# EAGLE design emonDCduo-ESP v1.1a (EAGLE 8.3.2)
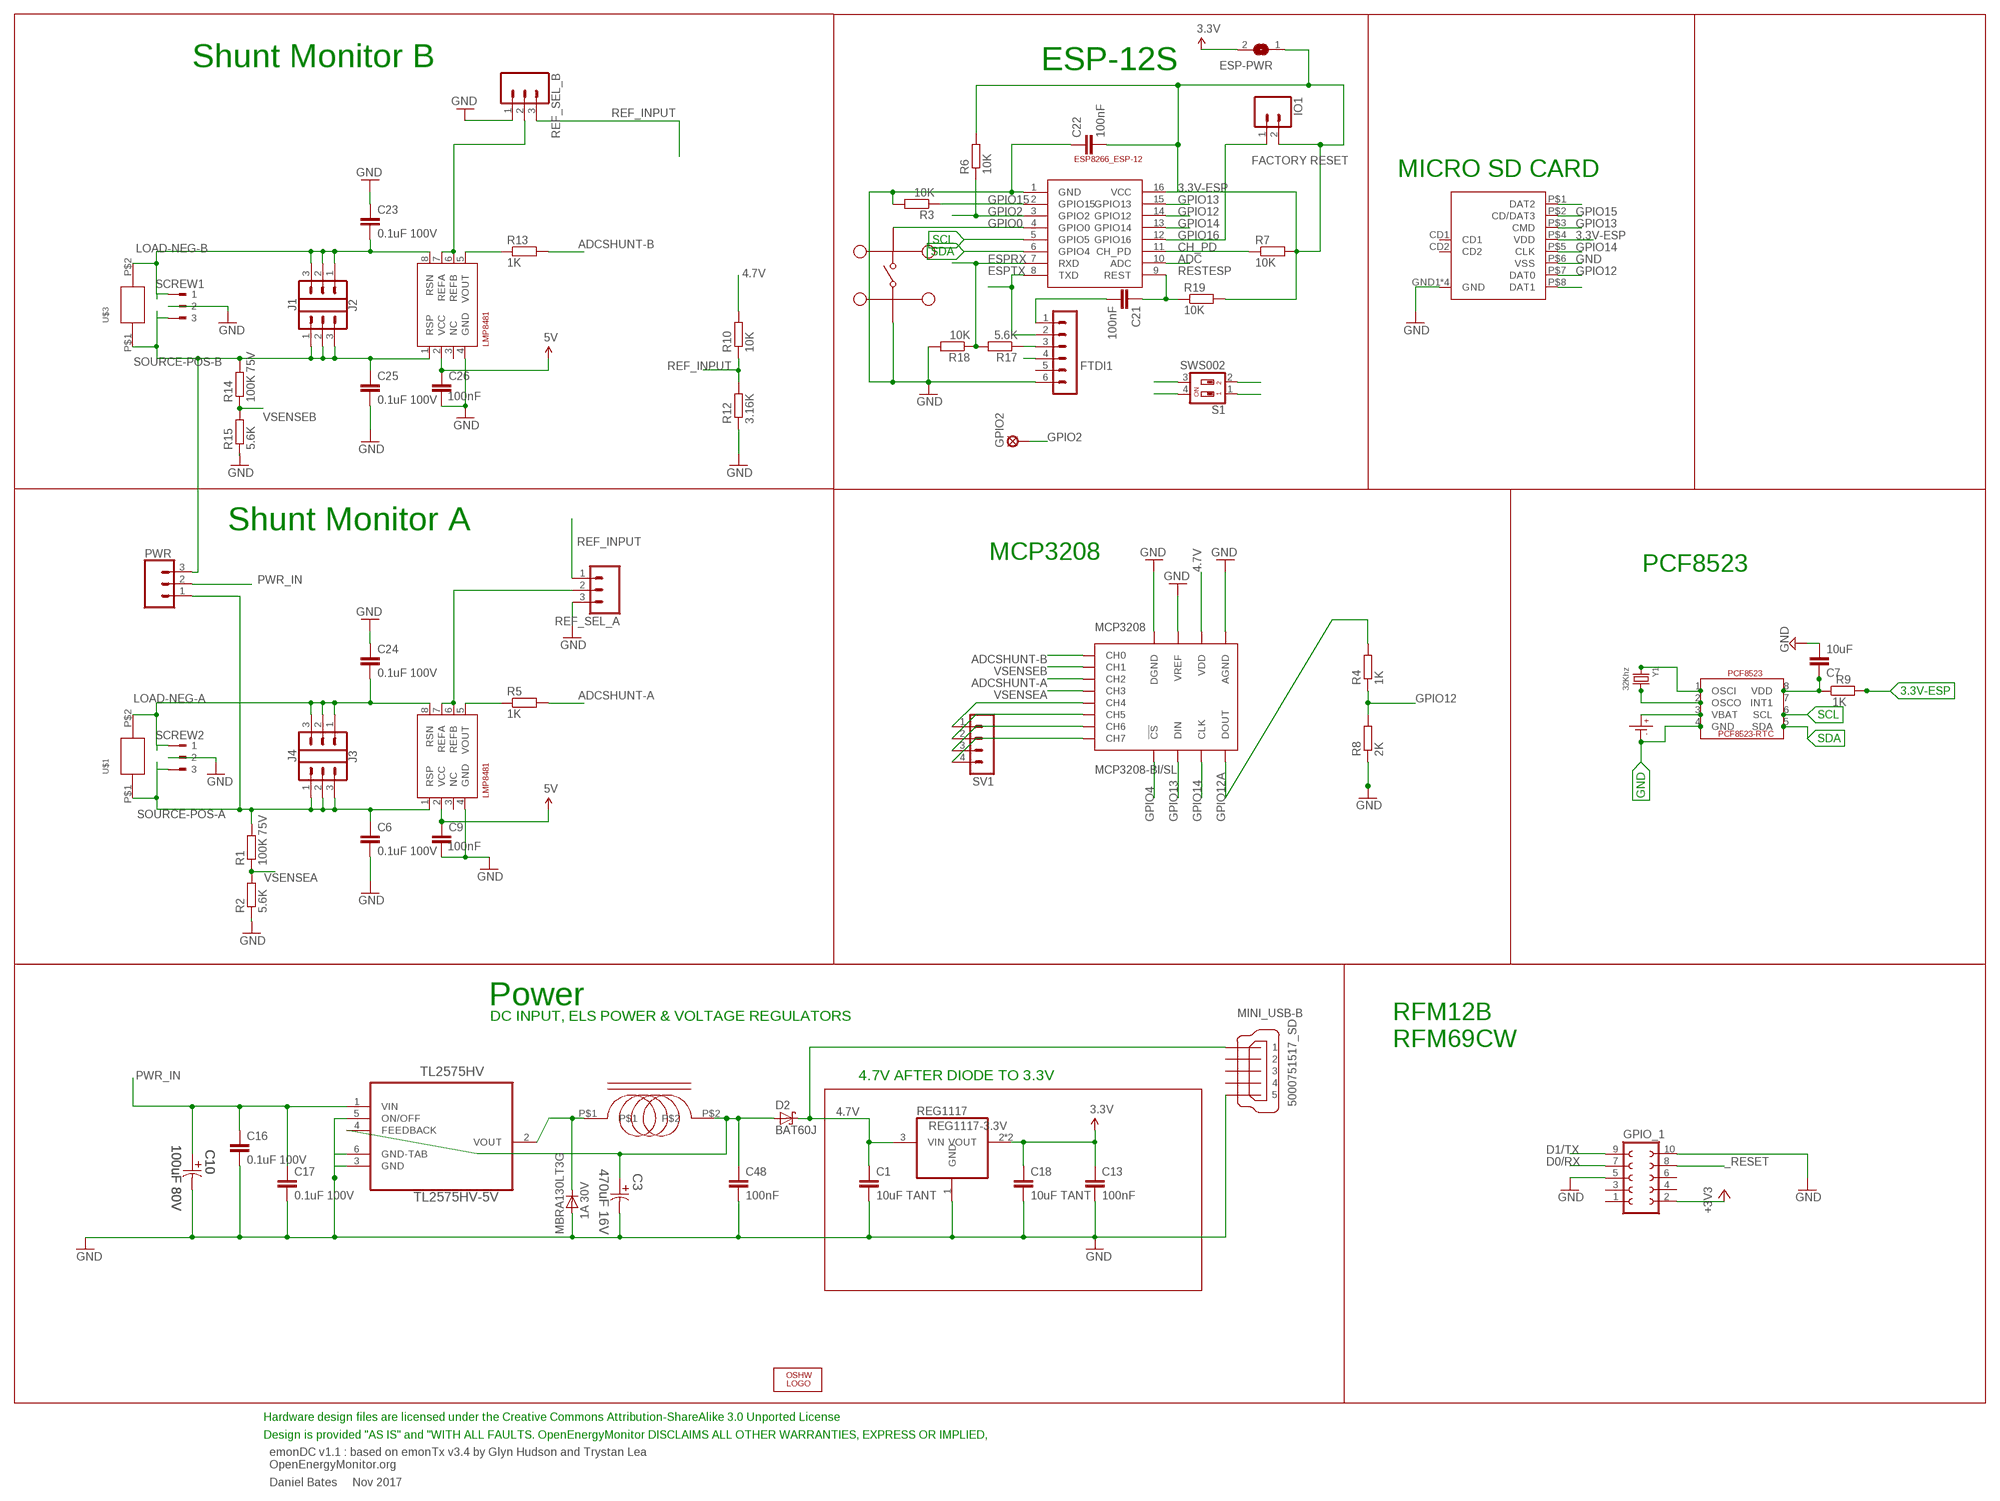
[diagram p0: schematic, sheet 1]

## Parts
C1  10uF TANT  C-EUC0603  [C0603]
C3  470uF 16V  EEE-FK1C471P-CASE-F  [CAPAE830X1050N]
C6  0.1uF 100V  C-EUC0603  [C0603]
C7  10uF  C-EUC0603  [C0603]
C9  100nF  C-EUC0603  [C0603]
C10  100uF 80V  EEV-FK1K101Q-CASE-H13  [CAPAE1350X1400N]
C13  100nF  C-EUC0603  [C0603]
C16  0.1uF 100V  C-EUC0603  [C0603]
C17  0.1uF 100V  C-EUC0603  [C0603]
C18  10uF TANT  C-EUC0603  [C0603]
C21  100nF  C-EUC0603  [C0603]
C22  100nF  C-EUC0603  [C0603]
C23  0.1uF 100V  C-EUC0603  [C0603]
C24  0.1uF 100V  C-EUC0603  [C0603]
C25  0.1uF 100V  C-EUC0603  [C0603]
C26  100nF  C-EUC0603  [C0603]
C48  100nF  C-EUC0603  [C0603]
D1  MBRA130LT3G  [DO-214]
D2  BAT60J  [SOD323_ST]
ESP-12  ESP8266_ESP-12  [ESP8266-ESP12]
ESP-PWR  SJ  [SJ]
FTDI1  FTDI-ESP  MA06-1  [MA06-1]
GPIO2  LSP11  [LSP11]
GPIO_1  FE05-2  [FE05-2]
I1  330uH  SRR0603-331KL  [SRR0603-331KL]
IO1  M02PTH  [1X02]
J1  CONN_03  [1X03]
J2  CONN_03  [1X03]
J3  CONN_03  [1X03]
J4  CONN_03  [1X03]
LOGO1  OSHW_LOGO_6MILX0200-NT  [OSHW_6X200_NOTEXT]
MC2  MC32882  [SWITCH_TACT_MULTICOMP]
MCP3208  MCP3208-BI/SL  [SOIC16]
MINI_USB-B  5000751517_SD  [5000751517_SD]
PCF8523  PCF8523_RTC  [SOIC_8]
PWR  CONN_03  [1X03]
R1  100K 75V  R-EU_R0603  [R0603]
R2  5.6K  R-EU_R0603  [R0603]
R3  10K  R-EU_R0603  [R0603]
R4  1K  R-EU_R0603  [R0603]
R5  1K  R-EU_R0603  [R0603]
R6  10K  R-EU_R0603  [R0603]
R7  10K  R-EU_R0603  [R0603]
R8  2K  R-EU_R0603  [R0603]
R9  1K  R-EU_R0603  [R0603]
R10  10K  R-EU_R0603  [R0603]
R12  3.16K  R-EU_R0603  [R0603]
R13  1K  R-EU_R0603  [R0603]
R14  100K 75V  R-EU_R0603  [R0603]
R15  5.6K  R-EU_R0603  [R0603]
R17  5.6K  R-EU_R0603  [R0603]
R18  10K  R-EU_R0603  [R0603]
R19  10K  R-EU_R0603  [R0603]
REF_SEL_A  2212S-02SG-85  CONN_03  [1X03]
REF_SEL_B  2212S-02SG-85  CONN_03  [1X03]
REG1117  REG1117-3.3V  REG1117-VOUT4  [SOT223]
S1  SWS002  [SMS-002]
SCREW1  180-3  [180-3]
SCREW2  180-3  [180-3]
SHUNTMON-A  LMP8481  LMP8481-H  [S-PDSO-G08]
SHUNTMON-B  LMP8481  LMP8481-H  [S-PDSO-G08]
SV1  MA04-1  [MA04-1]
TL2575HV  TL2575HV-5V  TL2575HV-05IKTTR  [TO-263]
U$1  EBW_SERIES_10.5MM  [EBW_SERIES_10.5MM]
U$2  MOLEX_MICRO_SD_1040310811  [MOLEX_MICROSD_EXPOSED]
U$3  EBW_SERIES_10.5MM  [EBW_SERIES_10.5MM]
U$18  CR1220SMD  [CR1220SMD]
Y1  32Khz  CRYSTAL8X3.8SMT  [CRYSTAL_8X3.8]

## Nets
3.3V: C13.1 C18.1 ESP-PWR.2 GPIO_1.2 REG1117.2(VOUT) REG1117.4(VOUT) ; supply symbol labelled +3V3
3.3V-ESP: C22.2 ESP-12.16(VCC) ESP-PWR.1 IO1.2 R6.2 R7.2 R9.2 R19.2 U$2.P$4(VDD)
4.7V [power]: C1.1 C9.1 C26.1 D2.C FTDI1.4 MCP3208.16(VDD) MINI_USB-B.VBUS R10.2 REG1117.3(VIN) SHUNTMON-A.2(VCC) SHUNTMON-B.2(VCC) ; supply symbol labelled 5V
5.0V [power]: C3.1 C48.1 D2.A I1.P$2 TL2575HV.4(FEEDBACK)
_RESET: GPIO_1.8
ADC: ESP-12.10(ADC)
ADCSHUNT-A: MCP3208.3(CH2) R5.2
ADCSHUNT-B: MCP3208.1(CH0) R13.2
CH_PD: ESP-12.11(CH_PD) R7.1
D0/RX: GPIO_1.7 S1.2
D1/TX: GPIO_1.9 S1.1
ESPRX: ESP-12.7(RXD) R17.2 R18.1 S1.4
ESPTX: ESP-12.8(TXD) FTDI1.2 S1.3
GND [thin_power]: C1.2 C3.2 C6.2 C7.2 C9.2 C10.2 C13.2 C16.2 C17.2 C18.2 C22.1 C23.1 C24.1 C25.2 C26.2 C48.2 D1.P$2(A) ESP-12.1(GND) FTDI1.6 GPIO_1.5 GPIO_1.10 MC2.P$1 MC2.P$2 MCP3208.9(DGND) MCP3208.14(AGND) MCP3208.15(VREF) MINI_USB-B.GND1 MINI_USB-B.GND2 MINI_USB-B.GND3 PCF8523.4(GND) R2.1 R3.2 R8.1 R12.1 R15.1 R18.2 REF_SEL_A.3 REF_SEL_B.1 REG1117.1(GND) SCREW1.2 SCREW2.2 SHUNTMON-A.4(GND) SHUNTMON-B.4(GND) TL2575HV.3(GND) TL2575HV.5(ON/OFF) TL2575HV.6(GND-TAB) U$2.GND1(GND) U$2.GND2(GND) U$2.GND3(GND) U$2.GND4(GND) U$2.P$6(VSS) U$18.P-(P$-)
GPIO0: ESP-12.4(GPIO0) MC2.P$3 MC2.P$4
GPIO2: ESP-12.3(GPIO2) GPIO2.MP R6.1
GPIO4: MCP3208.10(!CS)
GPIO12: ESP-12.14(GPIO12) R4.1 R8.2 U$2.P$7(DAT0)
GPIO12A: MCP3208.12(DOUT) R4.2
GPIO13: ESP-12.15(GPIO13) MCP3208.11(DIN) U$2.P$3(CMD)
GPIO14: ESP-12.13(GPIO14) MCP3208.13(CLK) U$2.P$5(CLK)
GPIO15 [thin_power]: ESP-12.2(GPIO15) R3.1 U$2.P$2(CD/DAT3)
GPIO16: ESP-12.12(GPIO16) IO1.1
IND: D1.P$1(C) I1.P$1 TL2575HV.2(VOUT)
LOAD-NEG-A: C24.2 J4.1 J4.2 J4.3 SCREW2.1 SHUNTMON-B.8(RSN) U$1.P$2
LOAD-NEG-B: C23.2 J1.1 J1.2 J1.3 SCREW1.1 SHUNTMON-A.8(RSN) U$3.P$2
N$1: MCP3208.5(CH4) SV1.1
N$3: MCP3208.6(CH5) SV1.2
N$4: R13.1 SHUNTMON-A.5(VOUT)
N$5: MCP3208.7(CH6) SV1.3
N$6: R5.1 SHUNTMON-B.5(VOUT)
N$7: U$2.P$1(DAT2)
N$9: MCP3208.8(CH7) SV1.4
N$10: C7.1 PCF8523.8(VDD) R9.1
N$30: C21.2 FTDI1.1
N$32: U$2.P$8(DAT1)
N$36: FTDI1.3 R17.1
N$43: PCF8523.3(VBAT) U$18.P+(P$+)
N$44: PCF8523.2(OSCO) Y1.P$4
N$45: PCF8523.1(OSCI) Y1.P$1
PWR_IN: C10.1 C16.1 C17.1 PWR.2 TL2575HV.1(VIN)
REF_A_INPUT [thin_power]: REF_SEL_A.2 SHUNTMON-B.6(REFB) SHUNTMON-B.7(REFA)
REF_B_INPUT: REF_SEL_B.2 SHUNTMON-A.6(REFB) SHUNTMON-A.7(REFA)
REF_INPUT: R10.1 R12.2 REF_SEL_A.1 REF_SEL_B.3
RESTESP: C21.1 ESP-12.9(REST) R19.1
SCL: ESP-12.5(GPIO5) PCF8523.6(SCL)
SDA: ESP-12.6(GPIO4) PCF8523.5(SDA)
SOURCE-POS-A: C6.1 J3.1 J3.2 J3.3 PWR.1 R1.2 SCREW2.3 SHUNTMON-B.1(RSP) U$1.P$1
SOURCE-POS-B: C25.1 J2.1 J2.2 J2.3 PWR.3 R14.2 SCREW1.3 SHUNTMON-A.1(RSP) U$3.P$1
VSENSEA: MCP3208.4(CH3) R1.1 R2.2
VSENSEB: MCP3208.2(CH1) R14.1 R15.2
Unconnected: FTDI1.5 GPIO_1.1 GPIO_1.3 GPIO_1.4 GPIO_1.6 MINI_USB-B.D+ MINI_USB-B.D- MINI_USB-B.ID PCF8523.7(INT1) SHUNTMON-A.3(NC) SHUNTMON-B.3(NC) U$2.CD1 U$2.CD2

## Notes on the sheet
- Shunt Monitor B | ESP-12S
- FACTORY RESET
- MICRO SD CARD
- Shunt Monitor A
- MCP3208
- PCF8523
- Power
- DC INPUT, ELS POWER & VOLTAGE REGULATORS
- RFM12B
  RFM69CW
- 4.7V AFTER DIODE TO 3.3V
- Hardware design files are licensed under the Creative Commons Attribution-ShareAlike 3.0 Unported License
- Design is provided "AS IS" and "WITH ALL FAULTS. OpenEnergyMonitor DISCLAIMS ALL OTHER WARRANTIES, EXPRESS OR IMPLIED,
- emonDC v1.1 : based on emonTx v3.4 by Glyn Hudson and Trystan Lea
  OpenEnergyMonitor.org
- Daniel Bates     Nov 2017

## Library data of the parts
C1 C7 C13 C16-C18 C21 C22 C48 = rcl:C-EU: CAPACITOR, European symbol
C3 = Panasonic-EEEFK_EEEFP:EEE-: Aluminum Electrolytic Capacitors,Surface Mount Type; MPN: EEE-FK1C471P; OC_FARNELL: 9695710; OC_NEWARK: 96K9385; PACKAGE: CASE-F; SUPPLIER: PANASONIC; TOLERANCE: ±20 %; VALUE: 470UF; VOLTAGERATING: 16V
C6 C9 C23-C26 = rcl:C-EU: CAPACITOR, European symbol; MPN: C1608X7S2A104K080AB
C10 = Panasonic-EEE-EEV-EEF-ECQ:EEV-: Aluminum Electrolytic Capacitors,Surface Mount Type; MPN: EEVFK1K101Q; OC_FARNELL: 9696113; OC_NEWARK: 96K9484; SUPPLIER: PANASONIC; TOLERANCE: ±20 %; VALUE: 100UF; VOLTAGERATING: 80V
D1 = CASE 403D Diode:MBRA130LT3G: Fast switching diode; MF: ON SEMICONDUCTOR; MPN: MBRA130LT3G; OC_FARNELL: 9555978
D2 = diode:BAT60J: Schottky barrier diode
ESP-12 = ESP8266-ESP12:ESP8266_ESP-12
ESP-PWR = jumper:SJ: SMD solder JUMPER
FTDI1 = JeeLabs:MA06-1: PIN HEADER
GPIO2 = solpad:LSP11: SOLDER PAD
GPIO_1 = con-lsta:FE05-2: FEMALE HEADER; OC_FARNELL: unknown; OC_NEWARK: unknown
I1 = SRR0603-331KL:SRR0603-331KL: SRR0603-331KL; INDUCTANCE: 330uH; MF: BOURNS; MPN: SRR0603-331KL; OC_FARNELL: 2333890
IO1 = SparkFun:M02: Header 2
J1-J4 PWR = SparkFun-Connectors:CONN_03: Multi connection point. Often used as Generic Header-pin footprint for 0.1 inch spaced/style header connections On any of the 0.1 inch spaced packages, you can populate with these: Break Away Headers - Straight (PRT-00116) Break Away Male Headers - Right Angle (PRT-00553) Female Headers (PRT-00115)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
LOGO1 = ohw-logo:OSHW_LOGO_6MIL; OC_FARNELL: unknown
MC2 = multicomp tact switch:MC32882
MCP3208 = MCP3208:MCP3208
MINI_USB-B = 5000751517_sd:5000751517_SD
PCF8523 = IotaWatt_parts:PCF8523_RTC: PCF8523-RTC SOIC-8
R1 R14 = rcl:R-EU_: RESISTOR, European symbol; MPN: MCWR06X1003FTL
R2 R4 R8 R15 = rcl:R-EU_: RESISTOR, European symbol; MPN: MCWR06X5901FTL
R3 R5-R7 R9 R10 R12 R13 R17-R19 = rcl:R-EU_: RESISTOR, European symbol
REF_SEL_A REF_SEL_B = SparkFun-Connectors:CONN_03: Multi connection point. Often used as Generic Header-pin footprint for 0.1 inch spaced/style header connections On any of the 0.1 inch spaced packages, you can populate with these: Break Away Headers - Straight (PRT-00116) Break Away Male Headers - Right Angle (PRT-00553) Female Headers (PRT-00115)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; MF: MULTICOMP; MPN: 2212S-02SG-85; OC_FARNELL: 1593458
REG1117 = burr-brown:REG1117-VOUT4: 800mA and 1A Low Dropout (LDO) Positive Regulator 1.8V, 2.5V, 2.85V, 3.3V, 5V, and Adj; MF: TEXAS INSTRUMENTS; MPN: REG1117; OC_FARNELL: 1097566; OC_NEWARK: 14P6981
S1 = smd-special:SWS002: SMD Dip Switch 2 pol.
SCREW1 SCREW2 = con-weidmueller-sl35:180-3: WEIDMUELLER CLAMP CONNECTOR; OC_FARNELL: unknown; OC_NEWARK: unknown
SHUNTMON-A = lmp8481b:LMP8481: LMP8481MM-H/NOPB 100V/V; MF: TEXAS INSTRUMENTS; MPN: LMP8481MME-S/NOPB; OC_FARNELL: 2322044
SHUNTMON-B = lmp8481b:LMP8481: LMP8481MM-H/NOPB 100V/V; MF: TEXAS INSTRUMENTS; MPN: LMP8481MME-H/NOPB; OC_FARNELL: 2322044
SV1 = con-lstb:MA04-1: PIN HEADER; OC_FARNELL: unknown; OC_NEWARK: unknown
TL2575HV = TL2575HV:TL2575HV; MF: TEXAS INSTRUMENTS; MPN: LM2575HVS-15/NOPB; OC_FARNELL: 2492609
U$1 U$3 = EBW series shunt:EBW_SERIES_10.5MM
U$2 = MOLEX MICRO SD [exposed pins]:MOLEX_MICRO_SD_1040310811
U$18 = IotaWatt_parts:CR1220SMD: CR1220 Battery SMD
Y1 = microbuilder:CRYSTAL: Crystals

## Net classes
2 thin_power: width 0.254 mm

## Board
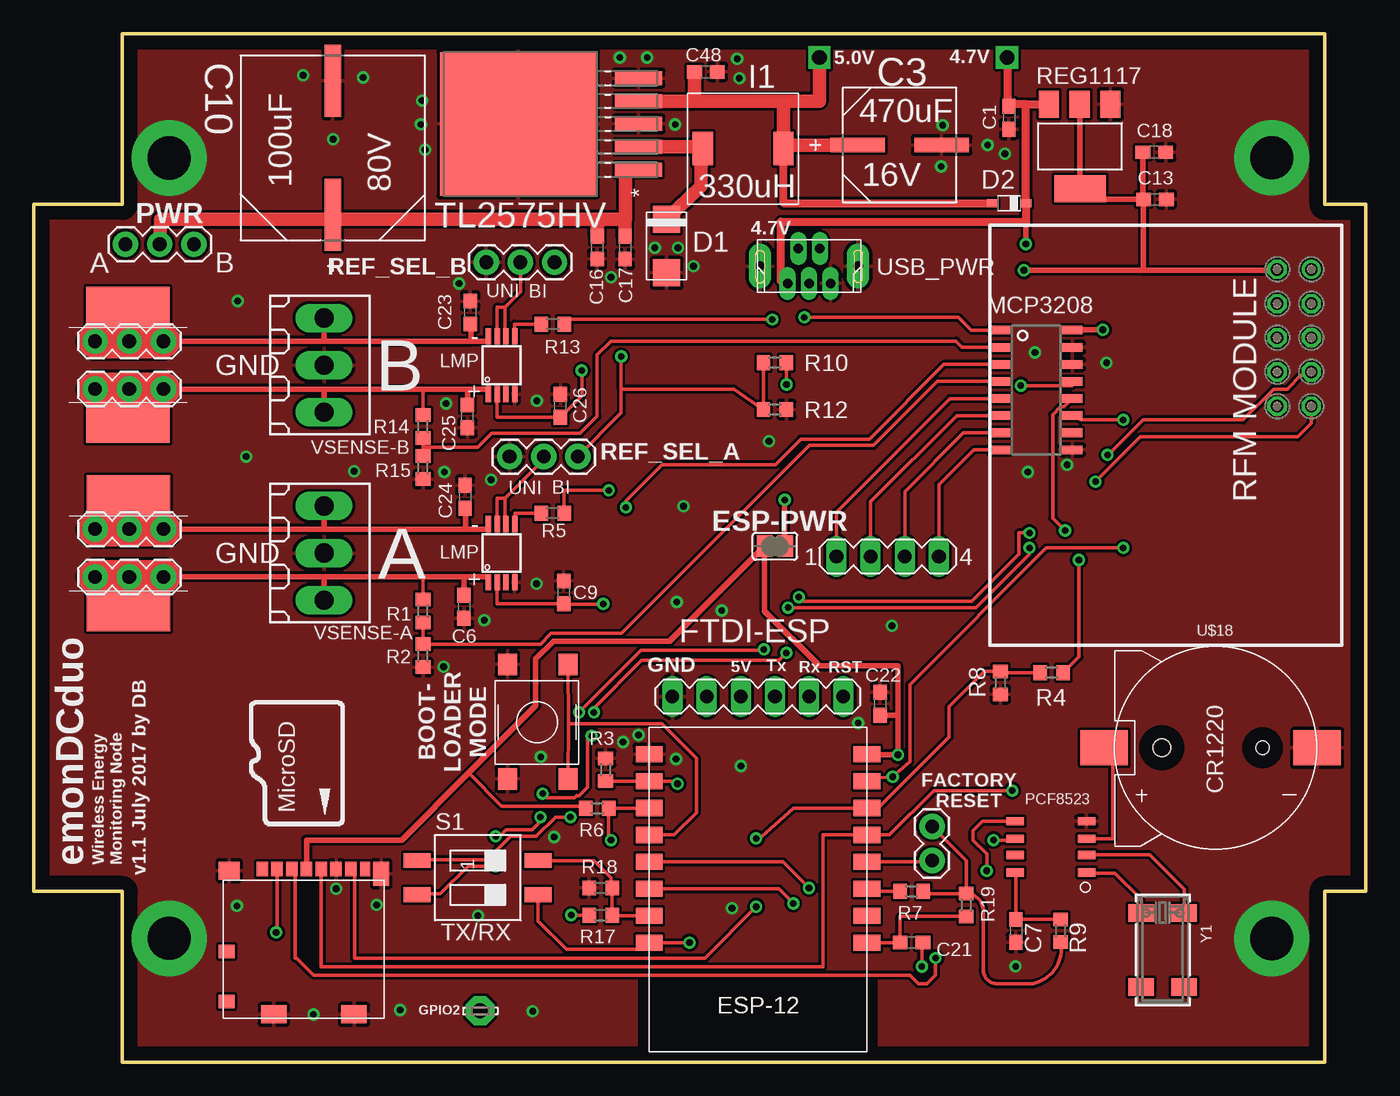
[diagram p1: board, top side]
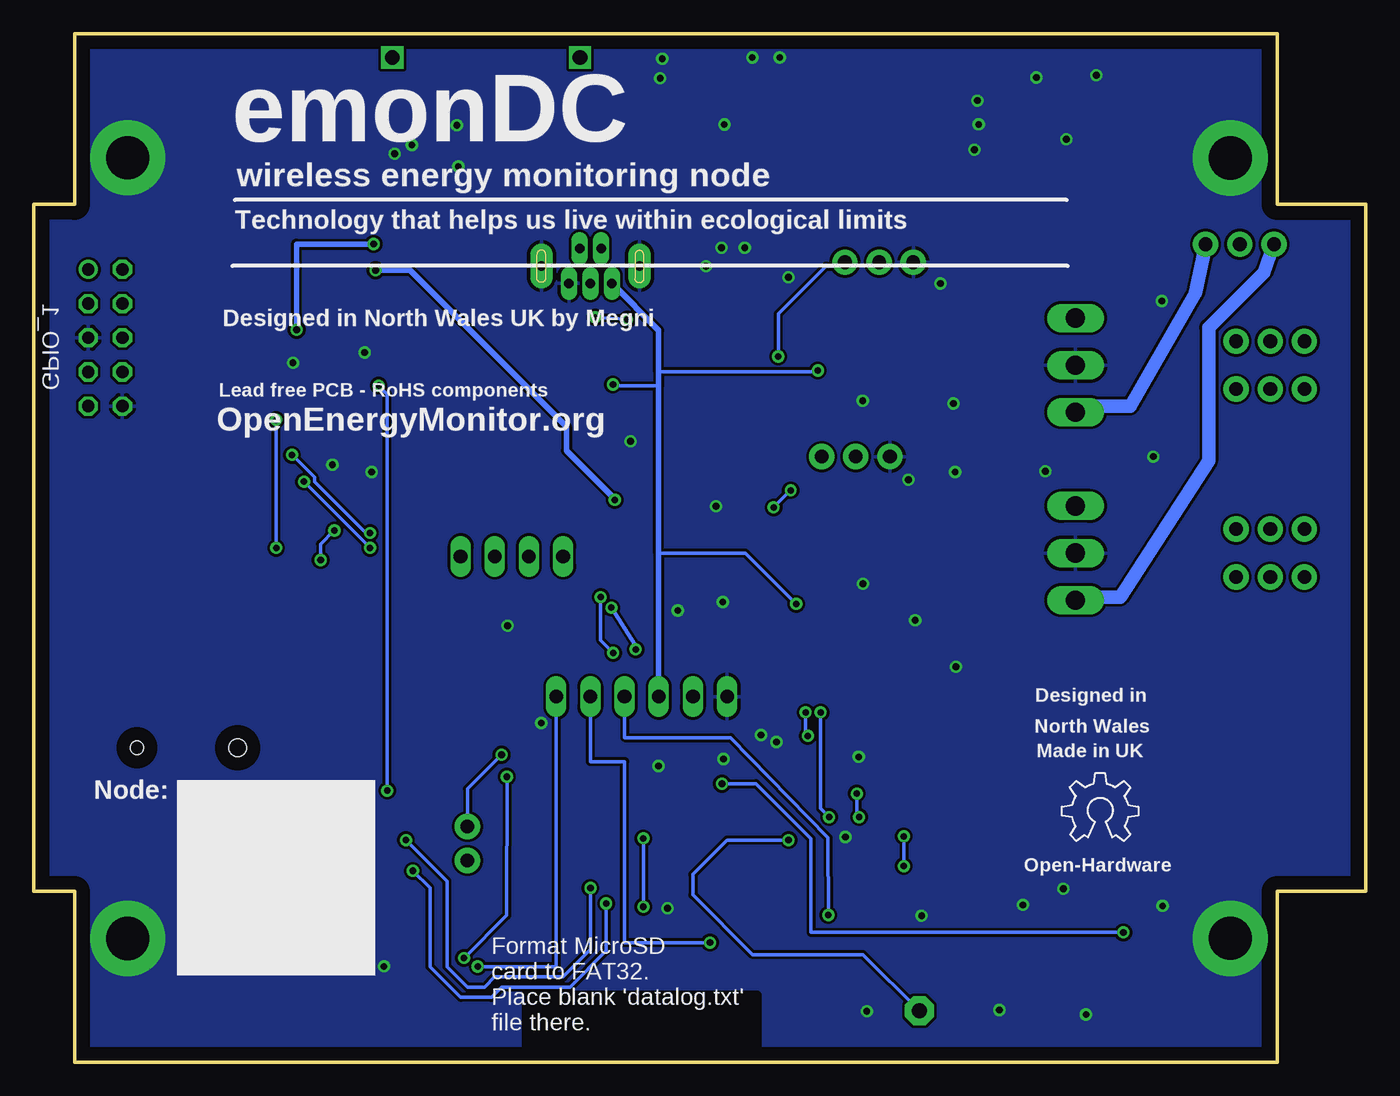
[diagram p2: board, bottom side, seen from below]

Size 99.06 x 76.45 mm. Coordinates in mm from the lower left corner, seen from the top.
Outline: 6.6,63.75 6.6,76.45 96.01,76.45 96.01,63.75 99.06,63.75 99.06,12.7 96.01,12.7 96.01,0 6.6,0 6.6,12.7 0,12.7 0,63.75 6.6,63.75
Copper layers (1*16): Top 0.035mm / dielectric 1.5mm / Bottom 0.035mm
Design rules "default *": minimum track width 10mil, minimum drill 19mil, track to track 8mil, track to pad 8mil, pad to pad 8mil, via to via 8mil, smd to smd 8mil, copper to edge 40mil, drill to drill 8mil, minimum pad ring 10mil, minimum via ring 8mil, stop-mask expansion 4mil, vias tented up to drill 0mil, thermal gap 10mil
tRestrict: area 45.2,1 to 62.5,6.1
bRestrict: area 45.2,1 to 62.5,5.1

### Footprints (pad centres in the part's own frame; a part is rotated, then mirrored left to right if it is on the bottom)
C0603 = smd 1.1 x 1: 1 -0.85,0; 2 0.85,0
CAPAE830X1050N = smd 4.064 x 1.092: 1 -3.124,0; 2 3.124,0
CAPAE1350X1400N = smd 5.359 x 1.194: 1 -4.978,0; 2 4.978,0
DO-214 = smd 2 x 2: P$1 -2,0; P$2 2,0
SOD323_ST = smd 0.8 x 0.6: A 1.25,0; C -1.25,0
ESP8266-ESP12 = smd 2 x 1.2: 1 16.2,2; 2 16.2,4; 3 16.2,6; 4 16.2,8; 5 16.2,10; 6 16.2,12; 7 16.2,14; 8 16.2,16; 9 0,16; 10 0,14; 11 0,12; 12 0,10; 13 0,8; 14 0,6; 15 0,4; 16 0,2
SJ = smd 1.168 x 1.6: 1 -0.762,0; 2 0.762,0
MA06-1 = drill 1.016 long: 1 0,0; 2 2.54,0; 3 5.08,0; 4 7.62,0; 5 10.16,0; 6 12.7,0
LSP11 = drill 1.118 pad 2.159 octagon: MP 0,0
FE05-2 = drill 0.914: 1 -5.08,1.27 | drill 0.914 octagon: 2 -5.08,-1.27; 3 -2.54,1.27; 4 -2.54,-1.27; 5 0,1.27; 6 0,-1.27; 7 2.54,1.27; 8 2.54,-1.27; 9 5.08,1.27; 10 5.08,-1.27
SRR0603-331KL = smd 1.5 x 2.5: P$1 -3,0; P$2 3,0
1X02 = drill 1.016 pad 1.88: 1 0,0; 2 2.54,0
1X03 = drill 1.016 pad 1.88: 1 0,0; 2 2.54,0; 3 5.08,0
SWITCH_TACT_MULTICOMP = smd 1.6 x 1.4: P$1 -1.1,5.3; P$2 7.4,5.3; P$3 -1.1,0.8; P$4 7.4,0.8
SOIC16 = smd 0.635 x 1.524: 1 -4.445,-2.695; 2 -3.175,-2.695; 3 -1.905,-2.695; 4 -0.635,-2.695; 5 0.635,-2.695; 6 1.905,-2.695; 7 3.175,-2.695; 8 4.445,-2.695; 9 4.445,2.695; 10 3.175,2.695; 11 1.905,2.695; 12 0.635,2.695; 13 -0.635,2.695; 14 -1.905,2.695; 15 -3.175,2.695; 16 -4.445,2.695
5000751517_SD = drill 0.7 pad 1.016 long: D+ 0,-1.3; D- -0.8,1.3; GND1 1.6,-1.3; ID 0.8,1.3; VBUS -1.6,-1.3 | drill 0.7 pad 1.676 long: GND2 3.65,0; GND3 -3.65,0
SOIC_8 = smd 1.3 x 0.6: 1 -2.6,1.9; 2 -2.6,0.6; 3 -2.6,-0.6; 4 -2.6,-1.9; 5 2.7,-1.9; 6 2.7,-0.6; 7 2.7,0.6; 8 2.7,1.9
R0603 = smd 1 x 1.1: 1 -0.85,0; 2 0.85,0
SOT223 = smd 1.499 x 2.007: 1 -2.261,-3.15; 2 0.025,-3.15; 3 2.311,-3.15 | smd 3.81 x 2.007: 4 0,3.15
SMS-002 = smd 1.092 x 2.007: 1 -1.27,-4.496; 2 1.27,-4.496; 3 1.27,4.496; 4 -1.27,4.496
180-3 = drill 1.422 long: 1 -3.5,0; 2 0,0; 3 3.5,0
S-PDSO-G08 = smd 0.4 x 1.2: 1 -0.975,-2.157; 2 -0.325,-2.157; 3 0.325,-2.157; 4 0.975,-2.157; 5 0.975,2.157; 6 0.325,2.157; 7 -0.325,2.157; 8 -0.975,2.157
MA04-1 = drill 1.016 long: 1 -3.81,0; 2 -1.27,0; 3 1.27,0; 4 3.81,0
TO-263 = smd 1.041 x 3.505: 1 -3.404,-8.788; 2 -1.702,-8.788; 3 0,-8.788; 4 1.702,-8.788; 5 3.404,-8.788 | smd 10.668 x 11.659: 6 0,0.152
EBW_SERIES_10.5MM = smd 3 x 6.2: P$1 -4.3,0; P$2 4.3,0
MOLEX_MICROSD_EXPOSED = smd 1.195 x 1.005: CD1 5.349,0.435; CD2 5.349,4.135 | smd 1.907 x 1.348: GND1 -4.112,5.104; GND2 1.853,5.104 | smd 1.17 x 1.793: GND3 -6.134,-5.352 | smd 1.551 x 1.348: GND4 5.167,-5.577 | smd 0.851 x 1.092: P$1 2.707,-5.703; P$2 1.617,-5.703; P$3 0.522,-5.699; P$4 -0.586,-5.701; P$5 -1.676,-5.703; P$6 -2.769,-5.703; P$7 -3.875,-5.701 | smd 0.749 x 1.092: P$8 -4.935,-5.701
CR1220SMD = smd 3.54 x 2.6: P+ 8.3,0; P- -7.55,0 | hole 1: -3.5,0 | hole 1.3: 4,0
CRYSTAL_8X3.8 = smd 1.3 x 1.9: P$1 -2.75,-1.6; P$2 2.75,-1.6; P$3 2.75,1.6; P$4 -2.75,1.6

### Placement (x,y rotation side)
C1  72.52,70.21 270 top
C3  64.39,68.17 0 top
C6  32,33.86 270 top
C7  73.04,9.76 270 top
C9  39.42,34.93 90 top
C10  22.25,67.96 90 top
C13  83.38,64.13 0 top
C16  41.9,60.55 270 top
C17  43.97,60.55 270 top
C18  83.32,67.64 0 top
C21  65.28,8.89 0 top
C22  62.94,26.64 270 top
C23  32.46,55.73 270 top
C24  32.08,42.04 270 top
C25  32.26,48.01 270 top
C26  39.17,48.8 90 top
C48  49.99,73.61 0 top
D1  47.06,60.67 270 top
D2  72.53,63.85 180 top
ESP-12  61.98,24.89 180 top
ESP-PWR  55.12,38.35 0 top
FTDI1  60.2,27.18 180 top
GPIO2  33.21,3.81 0 top
GPIO_1  93.73,53.85 270 top
I1  52.76,67.91 0 top
IO1  66.8,14.99 90 top
J1  4.57,53.59 0 top
J2  4.57,50.04 0 top
J3  4.57,36.07 0 top
J4  4.57,39.62 0 top
LOGO1  22.6,16.43 0 bottom
MC2  40.53,22.17 90 top
MCP3208  74.54,49.96 270 top
MINI_USB-B  57.66,59.18 0 top
PCF8523  75.69,16 180 top
PWR  6.84,60.8 0 top
R1  28.96,33.53 90 top
R2  28.96,30.23 90 top
R3  42.53,21.74 90 top
R4  75.69,28.96 0 top
R5  38.6,40.81 0 top
R6  41.91,18.87 180 top
R7  65.28,12.7 0 top
R8  71.88,28.19 90 top
R9  76.36,9.77 270 top
R10  55.12,52 0 top
R12  55.12,48.51 180 top
R13  38.61,54.86 0 top
R14  28.96,47.24 90 top
R15  28.96,44.2 90 top
R17  42.16,10.92 0 top
R18  42.16,12.95 180 top
R19  69.34,11.68 90 top
REF_SEL_A  40.47,45.01 180 top
REF_SEL_B  33.65,59.46 0 top
REG1117  77.8,68.07 180 top
S1  33.02,13.72 270 top
SCREW1  21.59,51.82 270 top
SCREW2  21.59,37.85 270 top
SHUNTMON-A  34.8,51.82 0 top
SHUNTMON-B  34.8,37.85 0 top
SV1  63.5,37.59 0 top
TL2575HV  36.19,69.74 90 top
U$1  7.05,37.82 90 top
U$2  19.71,8.66 180 top
U$3  7.02,51.83 90 top
U$18  87.88,23.37 180 top
Y1  83.95,8.35 270 top

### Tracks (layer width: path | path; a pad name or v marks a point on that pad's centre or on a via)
3.3V  (via drill 0.5)
  Top 0.254: 55.94,38.39 ESP-PWR.2 | 92.46,58.86 GPIO_1.2
  Top 0.406: REG1117.2 77.76,71.22 | 82.51,58.86 92.46,58.86 | 82.51,58.86 v73.63,58.86 | REG1117.4 78.6,64.13 C13.1 | C13.1 82.47,64.18 C18.1 | C13.1 82.51,64.11 82.51,58.86 | v55.84,41.8 55.84,38.49 55.94,38.39
  Bottom 0.406: v73.63,58.86 71.06,58.86 59.44,47.24 59.44,45.45 55.87,41.89 55.87,41.83 v55.84,41.8
3.3V-ESP  (via drill 0.5)
  Top 0.254: R7.2 66.13,12.53 R19.2 | R6.2 40.89,19.04 34.81,19.04 32.35,21.5 | IO1.2 69.34,14.99 R19.2 | R19.2 arc-90 70.61,11.26 70.61,6.86 arc90 71.63,5.84 74.29,5.84 arc90 R9.2
  Top 0.406: 64.26,25.91 64.26,29.46 58.42,29.46 54.36,33.53 ESP-PWR.1 47.29,31.28 38.65,31.28 37.34,29.97 37.34,26.49 32.35,21.5 27.35,16.51 20.3,16.51 U$2.P$4 | 64.26,25.91 v64.26,22.86 62.01,22.86 ESP-12.16 | C22.2 64.15,25.8 64.26,25.91
  Bottom 0.254: v64.26,22.86 66.8,20.32 IO1.2
4.7V  (via drill 0.5, 1.1)
  Top 0.254: SHUNTMON-A.2 34.47,47.95 C26.1 40.76,49.54 40.76,51.36 40.75,51.36 v40.75,51.41 | SHUNTMON-B.2 34.47,34.08 C9.1 39.46,34.04 42.42,34.04 42.39,34.07 v42.36,34.07 | R10.2 55.98,51.98 v55.98,50.38
  Top 0.406: D2.C 73.96,63.85 | 72.39,71.06 C1.1 72.52,71.22 | 73.78,62.48 73.79,62.48 v73.79,60.81 | v79.5,54.44 77.27,54.44 MCP3208.16 | MINI_USB-B.VBUS 55.86,58.08 55.56,58.08
  Top 0.61: v72.39,74.68 72.39,71.06 | 73.78,71.22 D2.C 73.78,62.48 55.56,62.48 55.56,58.08 | 73.78,71.22 REG1117.3 | 73.78,71.22 72.52,71.22
  Bottom 0.254: v55.98,50.38 55.9,50.29 52.58,50.29 | v40.75,51.41 40.85,51.31 52.58,51.31 | v42.36,34.07 46.14,37.85 52.58,37.85
  Bottom 0.406: v79.5,54.44 79.5,60.81 v73.79,60.81 | FTDI1.4 52.58,37.85 52.58,50.29 52.58,51.31 52.58,54.4 MINI_USB-B.VBUS
5.0V  (via drill 1.1)
  Top 0.61: D2.A 55.76,63.85 I1.P$2
  Top 1.016: TL2575HV.4 49.14,71.44 | 49.14,71.44 C48.1 | 55.76,71.44 I1.P$2 55.5,68.17 C3.1 | 55.76,71.44 49.14,71.44 | v58.42,74.68 58.42,71.44 55.76,71.44
ADCSHUNT-A  (via drill 0.48)
  Top 0.254: v42.77,42.51 39.43,42.51 39.43,40.93 R5.2 | v44.04,41.24 44.04,41.72 46.74,44.42 55.15,44.42 57.05,46.32 62.14,46.32 67.69,51.88 71.82,51.88 MCP3208.3
  Bottom 0.254: v44.04,41.24 v42.77,42.51
ADCSHUNT-B  (via drill 0.48)
  Top 0.254: v57.31,55.37 68.77,55.37 69.72,54.42 71.82,54.42 MCP3208.1 | R13.2 39.43,54.9 39.43,55.21 54.99,55.21 v54.92,55.21
  Bottom 0.254: v54.92,55.21 v57.31,55.37
CH_PD
  Top 0.254: ESP-12.11 61.98,12.7 R7.1
D0/RX  (via drill 0.48)
  Top 0.254: v34.35,14.57 32.29,14.57 30.23,12.51 28.64,12.51 S1.2 | v34.35,16.8 34.67,16.8 35.15,17.27 37.05,17.27 37.69,17.91 v37.69,18.23 | v37.85,19.97 38.16,19.65 40.23,19.65 40.39,19.81 40.55,19.81 41.18,20.45 41.18,24.26 v41.5,24.26 | v41.66,26 41.66,26.32 45.21,29.88 55.42,29.88 v55.97,30.43 55.96,30.22 | v56.9,34.58 57.21,34.26 69.75,34.26 73.25,37.75 73.25,39.34 v74.04,39.34 | v79.85,45.15 79.66,44.89 82.52,47.75 89.92,47.75 92.2,50.04 93.22,50.04 94.23,51.05 94.8,51.05 95,51.25 GPIO_1.7
  Bottom 0.254: v34.35,16.8 v34.35,14.57 | v37.69,18.23 37.85,18.38 v37.85,19.97 | v41.5,24.26 41.66,24.42 v41.66,26 | v74.04,39.34 74.36,39.34 78.17,43.15 78.17,43.47 v79.85,45.15 | v55.97,30.43 56.9,31.35 v56.9,34.58
D1/TX  (via drill 0.48)
  Top 0.254: v39.91,18.23 38.8,18.23 37.37,16.8 35.47,16.8 33.72,15.05 28.64,15.05 S1.1 | v40.55,26 45.15,30.61 54.22,30.61 v54.29,30.68 | v56.1,33.78 70.07,33.78 74.04,37.75 v74.04,38.23 | v78.96,43.15 82.3,46.48 93.98,46.48 95,47.5 GPIO_1.9 95,48.7
  Bottom 0.254: v39.91,18.23 40.55,18.86 v40.55,26 | v54.29,30.68 54.32,31.02 v56.1,33.78 | v78.96,43.15 v74.04,38.23
ESPRX
  Top 0.254: ESP-12.7 42.79,10.89 R17.2 R18.1 42.93,13.04 42.93,13.72 41.66,14.99 S1.4
ESPTX  (via drill 0.5)
  Top 0.254: v48.77,8.89 ESP-12.8 45.27,8.38 39.62,8.38 37.52,10.49 S1.3
  Bottom 0.254: v48.77,8.89 55.12,8.89 55.12,22.35 57.66,22.35 FTDI1.2
GND  (via drill 0.5, 3.2 pad 5.59)
  Top 0.254: ESP-12.1 46.06,22.61
  Top 0.406: U$2.GND2 | U$2.P$6 22.48,14.39 | 25.86,13.97 25.91,13.97 25.96,14.02
  other vias: 10.08,67.21 92.07,67.23 52.47,73.15 10.08,9.2 92.07,9.2 33.51,32.85 15.17,56.58 30.55,43.87 37.41,49.17 70.94,68.18 30.66,48.96 37.39,35.57 47.77,22.53 51.93,11.44 22.49,12.89 42.93,58.34 49.07,59.16 67.59,69.65 47.7,69.7 28.88,71.47 20.04,73.36 24.49,73.2 15.81,45.01 30.48,29.4 34.01,43.3 20.81,3.54 47.92,60.54 44.98,24.32 25.51,11.7 61.31,25.22 15.12,11.62 38.69,16.74 31.64,57.88 23.83,43.93 43.83,23.8 37.71,22.7 33.04,10.88 27.25,3.88 37.11,3.79 46.19,60.53 67.48,66.58 72.22,67.52 52.32,74.58 29.11,67.83 28.79,69.71 43.59,74.69 45.62,74.69 22.27,68.6 48.33,41.33 47.82,34.21 51.17,33.58 63.82,32.44 52.6,22.02 73.93,43.87 79.77,52 74.44,52.76 76.85,44.42 54.68,46.15 73.01,7.12
  pour Bottom (isolate 0.127): 6.86,76.2 6.86,63.5 0.25,63.5 0.25,12.95 6.86,12.95 6.86,0.25 95.76,0.25 95.76,12.95 98.81,12.95 98.81,63.5 95.76,63.5 95.76,76.2
  pour Top (isolate 0.127): 6.86,76.2 6.86,63.5 0.25,63.5 0.25,12.95 6.86,12.95 6.86,0.25 95.76,0.25 95.76,12.95 98.81,12.95 98.81,63.5 95.76,63.5 95.76,76.2
GPIO0
  Top 0.254: MC2.P$3 39.77,25.15 | 39.77,25.15 MC2.P$4 | ESP-12.4 47.63,16.89 49.28,18.54 49.28,22.61 46.74,25.15 39.77,25.15
GPIO2  (via drill 0.5)
  Top 0.254: ESP-12.3 42.78,18.89 R6.1 42.76,16.68 v42.93,16.51
  Bottom 0.254: v42.93,16.51 47.5,16.51 50.04,13.97 50.04,12.45 45.6,8.01 37.4,8.01 GPIO2.MP
GPIO12  (via drill 0.5)
  Top 0.254: R4.1 71.97,28.96 R8.2 70.7,29.04 68.07,26.42 68.07,24.16 62.77,18.86 61.98,18.86 ESP-12.14 56.48,18.89 53.78,16.45 | 53.78,16.45 53.59,16.51 | v53.72,11.56 49.91,7.75 23.88,7.75 23.88,14.1 U$2.P$7 | v53.72,16.64 53.85,16.64 53.78,16.45
  Bottom 0.254: v53.72,16.64 v53.72,11.56
GPIO12A  (via drill 0.5)
  Top 0.254: 77.22,49.34 MCP3208.12 76.61,48.71 76.34,48.71 75.77,48.14 75.77,40.45 76.69,39.52 v76.7,39.52 | R4.2 77.72,30.14 v77.72,37.33
  Bottom 0.254: v76.7,39.52 77.72,38.5 v77.72,37.34 v77.72,37.33
GPIO13  (via drill 0.48, 0.5)
  Top 0.254: v67.06,7.75 67.06,6.48 66.42,5.84 65.79,5.84 65.15,6.48 20.83,6.48 19.56,7.75 19.43,7.75 19.43,14.1 U$2.P$3 | ESP-12.15 61.98,21.08 v63.87,21.22 65.15,22.35 65.15,28.07 75.31,38.23 v81.03,38.23 | v81.03,47.75 77.85,47.75 MCP3208.11
  Bottom 0.254: v67.06,7.75 63.88,10.92 v63.87,21.22 | v81.03,38.23 v81.03,47.75
GPIO14  (via drill 0.48)
  Top 0.254: U$2.P$5 21.39,7.11 58.67,7.11 58.67,16.89 ESP-12.13 63.63,16.89 66.93,20.19 v72.77,20.19 | v73.41,50.29 77.22,50.29 MCP3208.13
  Bottom 0.254: v73.41,50.29 72.77,49.66 v72.77,20.19
GPIO15  (via drill 0.5)
  Top 0.254: ESP-12.2 R3.1 47.88,20.89 v47.88,20.7 | v18.03,9.65 18.09,9.65 U$2.P$2
  Bottom 0.254: v47.88,20.7 45.35,20.7 41.25,16.6 41.25,9.65 v18.03,9.65
GPIO16
  Top 0.254: IO1.1 66.71,14.89 ESP-12.12
IND
  Top 1.016: TL2575HV.2 49.63,68.04 | 49.63,68.04 I1.P$1 | 49.63,68.04 49.63,65.1 D1.P$1
LOAD-NEG-A
  Top 0.406: 32.12,39.62 33.82,39.62 SHUNTMON-B.8 | C24.2 32.12,41.19 32.12,39.62 | J4.1 J4.2 J4.3 21.59,39.62 | 21.59,39.62 32.12,39.62 | SCREW2.1 21.59,39.62
  Top 2.54: J4.1 J4.3 9.68,39.6 | J4.2 7.11,42.06 U$1.P$2
LOAD-NEG-B
  Top 0.406: 32.51,53.59 33.82,53.59 SHUNTMON-A.8 | C23.2 32.51,54.88 32.51,53.59 | 9.68,53.57 J1.3 21.59,53.59 | 21.59,53.59 32.51,53.59 | SCREW1.1 21.59,53.59
  Top 2.54: J1.1 J1.2 | J1.2 J1.3 | U$3.P$2 7.02,53.69 J1.2
N$1
  Top 0.254: MCP3208.5 68.12,49.33 59.69,40.89 SV1.1
N$2
  Top 0.406: 77.72,64.9 77.8,64.9 77.8,71.15
N$3
  Top 0.254: MCP3208.6 68.63,48.06 62.23,41.66 SV1.2
N$4
  Top 0.254: SHUNTMON-A.5 35.77,54.86 R13.1
N$5
  Top 0.254: MCP3208.7 69.14,46.79 64.77,42.42 SV1.3
N$6
  Top 0.254: SHUNTMON-B.5 35.81,40.81 R5.1
N$9
  Top 0.254: MCP3208.8 69.9,45.52 67.31,42.93 SV1.4
N$10
  Top 0.254: R9.1 73.05,10.62 C7.1 73.04,14.06 PCF8523.8
N$30  (via drill 0.5)
  Top 0.254: v66.04,7.11 66.04,8.89 C21.2
  Bottom 0.254: FTDI1.1 60.2,7.11 v66.04,7.11
N$36  (via drill 0.5)
  Top 0.254: v39.97,10.94 R17.1
  Bottom 0.254: FTDI1.3 55.12,24.13 47.24,24.13 39.99,16.68 v39.97,10.94
N$43
  Top 0.254: PCF8523.3 80.26,16.6 80.26,23.11 79.58,23.11 U$18.P+
N$44
  Top 0.254: Y1.P$4 85.55,12.87 83.01,15.41 PCF8523.2
N$45
  Top 0.254: Y1.P$1 82.35,12.1 80.39,14.06 78.33,14.06 PCF8523.1
PWR_IN
  Top 1.016: 44.27,66.33 TL2575HV.1 44.01,66.33 44.01,62.66 43.94,62.66 | PWR.2 9.46,62.66 21.93,62.66 | 43.94,62.66 42.29,62.66 41.9,62.27 | C16.1 41.9,62.27 | C17.1 43.97,62.63 43.94,62.66 | 21.93,62.66 C10.1 | 41.9,62.27 41.9,62.66 21.93,62.66
REF_A_INPUT
  Top 0.254: REF_SEL_A.2 37.93,44.79 35.05,41.91 | 35.05,41.91 35.05,40.07 SHUNTMON-B.6 | SHUNTMON-B.7 34.47,41.91 35.05,41.91
REF_B_INPUT
  Top 0.254: 36.2,57.28 35.05,56.13 | 35.05,56.13 35.05,54.04 SHUNTMON-A.6 | REF_SEL_B.2 36.2,57.28 | 36.2,57.28 | SHUNTMON-A.7 34.47,56.13 35.05,56.13
REF_INPUT  (via drill 0.5)
  Top 0.254: 43.69,50.04 v43.69,52.45 | 43.69,50.04 43.69,48.26 40.47,45.04 REF_SEL_A.1 | R10.1 R12.2 52.07,50.04 43.69,50.04
  Bottom 0.254: v43.69,52.45 43.69,55.63 40.13,59.18 39.01,59.18 REF_SEL_B.3
RESTESP
  Top 0.254: ESP-12.9 C21.1 64.43,10.83 R19.1
SCL  (via drill 0.5)
  Top 0.254: ESP-12.5 55.72,14.89 v57.66,12.95 | v71.37,16.51 72.9,16.51 PCF8523.6
  Bottom 0.254: v57.66,12.95 57.66,8.38 59.69,6.35 64.77,6.35 65.53,5.59 66.8,5.59 68.33,7.11 68.33,13.46 v71.37,16.51
SDA  (via drill 0.5)
  Top 0.254: ESP-12.6 55.43,12.89 56.39,11.94 56.39,11.9 v56.49,11.8 | v70.87,14.22 70.87,15.49 69.85,16.51 69.85,17.21 70.55,17.91 72.98,17.91 PCF8523.5
  Bottom 0.254: v56.49,11.8 56.49,8.28 59.18,5.59 64.26,5.59 65.02,4.83 67.31,4.83 69.6,7.11 69.6,12.95 v70.87,14.22
SOURCE-POS-A
  Top 0.254: R1.2 28.96,36.07
  Top 0.406: 32,36.07 28.96,36.07 21.59,36.07 | 32,36.07 33.82,36.07 SHUNTMON-B.1 | C6.1 32,36.07 | J3.1 4.83,35.81 5.08,36.07 J3.2 J3.3 21.59,36.07 | SCREW2.3 21.59,36.07
  Top 2.54: J3.1 J3.3 9.68,36.1 | J3.2 7.11,33.58 U$1.P$1
  Bottom 1.016: PWR.1 7.6,58.7 11.68,54.61 11.68,44.7 18.26,34.57 21.62,34.57 SCREW2.3
SOURCE-POS-B
  Top 0.254: R14.2 28.96,50.04
  Top 0.406: 32.26,50.04 28.96,50.04 21.59,50.04 | 32.26,50.04 33.69,50.04 33.82,49.91 SHUNTMON-A.1 | C25.1 32.26,50.04 | J2.1 J2.2 J2.3 | J2.3 9.68,50.07 | 21.59,50.04 J2.3 | SCREW1.3 21.59,50.04
  Top 2.54: J2.1 J2.3 | J2.2 7.11,47.63 U$3.P$1
  Bottom 1.016: PWR.3 12.68,57.17 17.53,48.77 21.39,48.77 SCREW1.3
VSENSEA
  Top 0.254: R2.2 R1.1 | R2.2 37.69,31.08 38.48,31.88 43.72,31.88 57.69,45.85 62.45,45.85 67.21,50.61 71.82,50.61 MCP3208.4 | R2.2
VSENSEB
  Top 0.254: 28.96,44.96 R15.2 28.96,45.72 | R14.1 28.96,45.72 | MCP3208.2 69.03,53.14 68.58,53.59 42.93,53.59 41.91,52.58 41.91,48.01 40.64,46.74 34.04,46.74 33.02,45.72 28.96,45.72

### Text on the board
tPlace: VSENSE-B | VSENSE-A | MicroSD | TX/RX
bPlace: emonDC | wireless energy monitoring node | Technology that helps us live within ecological limits | Designed in North Wales UK by Megni | Lead free PCB - RoHS components | OpenEnergyMonitor.org | Designed in | North Wales | Made in UK | Node: | Open-Hardware | Format MicroSD / card to FAT32. / Place blank 'datalog.txt' / file there.
tNames: I1 | 470uF | 100uF | 16V | 80V | 330uH | D1 | USB_PWR | A | B | UNI | BI | B | GND | LMP | UNI | BI | A | GND | LMP | BOOT- / LOADER / MODE | FACTORY / RESET
tSilk: 5.0V | 4.7V | 4.7V | RFM MODULE | GND | 5V | Tx | Rx | RST | emonDCduo | Wireless Energy / Monitoring Node | v1.1 July 2017 by DB
_tsilk: Designed in | North Wales | Made in UK
_bsilk: SMT V0.6 rev3 | emonTx | wireless energy monitoring node | SMT V0.6 rev3 | emonTx | SMT V0.6 rev3 | emonTx | Technology that helps us live within ecological limits | wireless energy monitoring node | wireless energy monitoring node | Designed in North Wales UK by Glyn Hudson & Trystan Lea | Technology that helps us live within ecological limits | Technology that helps us live within ecological limits | Designed in North Wales UK by Glyn Hudson & Trystan Lea | 165mm ant | 433Mhz | Designed in North Wales UK by Glyn Hudson & Trystan Lea | 165mm ant | 165mm ant | 433Mhz | 433Mhz | 868Mhz | 82mm ant | 82mm ant | 82mm ant | 868Mhz | 868Mhz | 78mm ant | 915Mhz | 78mm ant | 915Mhz | 78mm ant | 915Mhz | 165mm ant | 433Mhz | 82mm ant | 868Mhz | 78mm ant | 915Mhz

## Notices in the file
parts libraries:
SparkFun-Connectors: Licensing: CC v3.0 Share-Alike You are welcome to use this library for commercial purposes.
SparkFun-Aesthetics: Licensing: Creative Commons ShareAlike 4.0 International - https://creativecommons.org/licenses/by-sa/4.0
